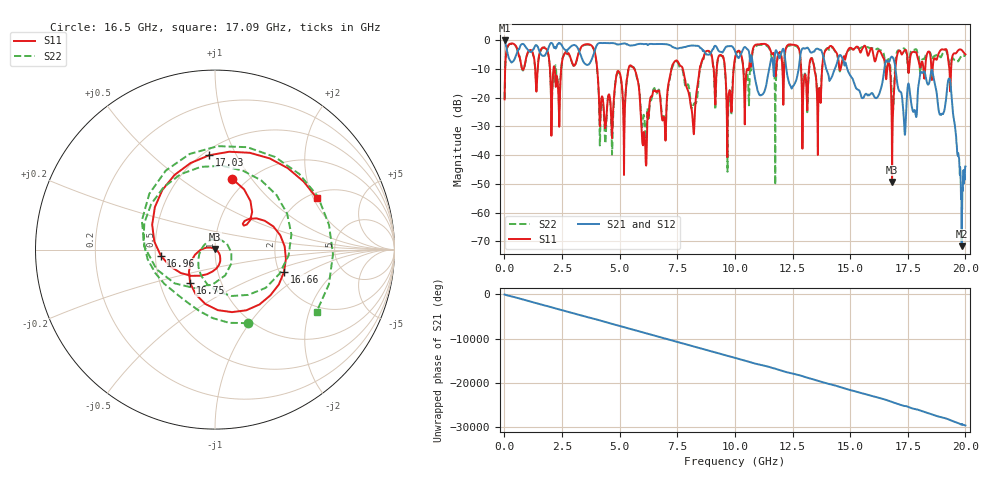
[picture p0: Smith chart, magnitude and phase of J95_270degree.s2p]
!Keysight Technologies,N5222A,MY51421036,A.10.65.16
!Date: Friday, March 31, 2023 14:18:35
!Correction: S11(Full 2 Port(1,2))
!S21(Full 2 Port(1,2))
!S12(Full 2 Port(1,2))
!S22(Full 2 Port(1,2))
!S2P File: Measurements: S11, S21, S12, S22:
# Hz S  dB  R 50
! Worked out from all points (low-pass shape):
!   2000 points, 10 MHz to 20 GHz, reference 50 ohm
!   highest |S21| = -0.13 dB at 10 MHz (marker M1); lowest = -71.7 dB at 19.84 GHz (marker M2)
!   |S21| within 3 dB of the highest: 1.897 GHz to 2.597 GHz (700.4 MHz wide, 31.2 % of centre); 3.945 GHz to 8.575 GHz (4.63 GHz wide, 74 % of centre)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
!   lowest |S11| = -49.4 dB at 16.82 GHz (marker M3), VSWR 1.01, Z = 49.9 + j0.323 ohm
!   |S11| at or under -10 dB: 4.026 GHz to 5.386 GHz (1.359 GHz wide, 28.9 % of centre); 5.633 GHz to 7.251 GHz (1.617 GHz wide, 25.1 % of centre); 7.739 GHz to 8.474 GHz (735 MHz wide, 9.07 % of centre)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
!   |S22| runs from -50.4 to -1.3 dB; largest |S21 - S12| = 0.015
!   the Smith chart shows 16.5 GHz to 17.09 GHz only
!   S11 on the Smith chart (normalised r, x): 16.5 GHz: 0.86, +0.81; 16.66 GHz: 2.12, -0.63; 16.75 GHz: 0.71, -0.28; 16.96 GHz: 0.54, -0.04; 17.03 GHz: 0.54, +0.78; 17.09 GHz: 2.20, +2.13
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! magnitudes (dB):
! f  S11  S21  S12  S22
! 10 MHz  -20.6  -0.1  -0.2  -20.5
! 3.35 GHz  -2.3  -6.1  -6.0  -2.4
! 4.37 GHz  -30.7  -1.0  -1.0  -35.4
! 5.61 GHz  -9.7  -1.8  -1.8  -9.5
! 6.08 GHz  -33.1  -1.4  -1.4  -27.7
! 6.68 GHz  -17.6  -1.4  -1.4  -17.4
! 8.19 GHz  -30.0  -1.9  -1.9  -22.8
! 8.85 GHz  -3.8  -5.1  -5.1  -4.1
! 9.76 GHz  -17.6  -2.1  -2.1  -19.5
! 10.01 GHz  -6.1  -3.9  -3.9  -6.5
! 13.34 GHz  -6.4  -4.3  -4.4  -6.3
! 16.5 GHz  -7.8  -9.0  -9.0  -6.9
! 16.66 GHz  -7.9  -7.6  -7.5  -6.6
! 16.67 GHz  -7.8  -7.6  -7.6  -6.6
! 16.75 GHz  -12.7  -6.3  -6.3  -10.1
! 16.82 GHz  -49.4  -5.8  -5.8  -20.8
! 16.96 GHz  -10.3  -9.6  -9.6  -8.1
! 17.03 GHz  -5.6  -14.4  -14.3  -4.2
! 17.09 GHz  -3.9  -16.9  -16.9  -3.6
! 19.3 GHz  -9.6  -13.4  -13.3  -7.5
! 19.84 GHz  -3.5  -71.7  -59.3  -5.7
! 20 GHz  -4.9  -44.0  -43.8  -5.7
